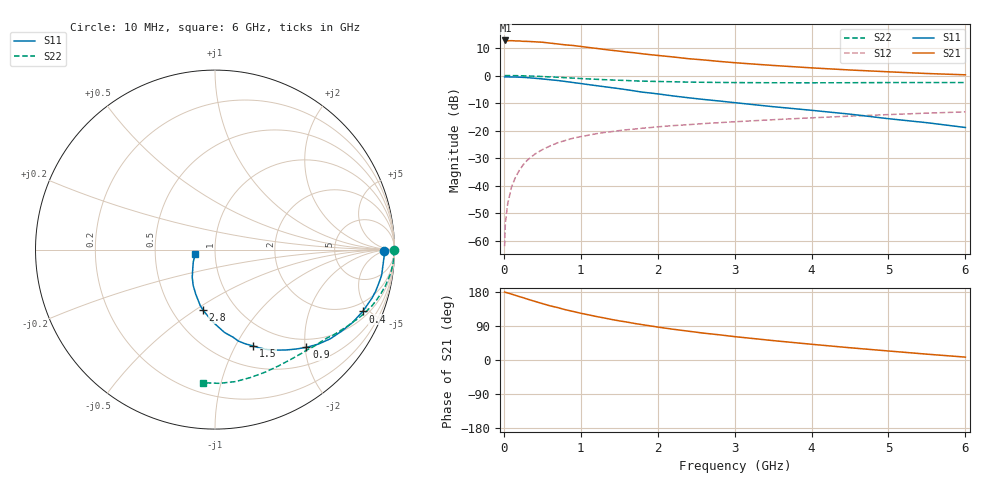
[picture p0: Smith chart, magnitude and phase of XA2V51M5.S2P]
! SIEMENS Discrete & RF Semiconductors
! BFY180
! Si NPN RF Bipolar Junction Transistor in MICRO-X
! VCE = 2.5 V  IC = 1.5 mA
! Common Emitter S-Parameters:  May  1997
# GHz  S  MA  R  50
!  f  S11  S21  S12  S22
! GHz  MAG  ANG  MAG  ANG  MAG  ANG  MAG  ANG
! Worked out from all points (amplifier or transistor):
!   36 points, 10 MHz to 6 GHz, reference 50 ohm
!   highest |S21| = 12.7 dB at 20 MHz (marker M1)
!   |S21| within 3 dB of that: start of sweep to 1.236 GHz
!   unconditionally stable (mu >= 1): 3.09 GHz to end of sweep
!   at 250 MHz: K = 0.11, MSG = 22.4 dB, |S12| = -32.5 dB
!   at 1.4 GHz: K = 0.62, MSG = 14.8 dB, |S12| = -20.4 dB
!   at 6 GHz: K = 1.07, MAG = 5.1 dB, |S12| = -13.2 dB
!   S11 on the Smith chart (normalised r, x): 10 MHz: 33, -5; 400 MHz: 1.36, -4.60; 900 MHz: 0.83, -2.03; 1.5 GHz: 0.73, -1.18; 2.8 GHz: 0.70, -0.54; 6 GHz: 0.80, -0.04
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0.01  0.9422 -0.5  4.269 179.3  0.0008 84.7  0.9964 -0.2
0.02  0.9449 -1.1  4.325 178.6  0.0021 104.7  0.9975 -0.6
0.05  0.9424 -2.7  4.265 177.0  0.0047 88.4  0.996 -1.5
0.1  0.9396 -5.8  4.283 173.9  0.0095 88.2  0.996 -3.1
0.15  0.9395 -8.7  4.247 170.7  0.0141 84.7  0.9945 -4.6
0.25  0.925 -14.4  4.173 164.5  0.0238 80.7  0.9879 -7.6
0.4  0.8925 -22.7  4.093 154.9  0.0372 75.1  0.9711 -11.9
0.5  0.8665 -28.1  4.016 148.9  0.0451 71.5  0.957 -14.7
0.6  0.8387 -32.9  3.872 143.0  0.0526 68.9  0.9438 -17.2
0.8  0.779 -42.6  3.595 132.7  0.0663 62.8  0.9123 -21.9
0.9  0.7458 -46.9  3.506 128.1  0.0728 59.8  0.8971 -24.1
1.1  0.6839 -54.9  3.227 119.2  0.0825 55.6  0.8665 -27.9
1.2  0.6551 -58.7  3.11 114.9  0.0878 53.8  0.8538 -29.8
1.5  0.5775 -68.4  2.768 103.3  0.1001 48.8  0.82 -34.7
1.8  0.4986 -78.3  2.48 93.2  0.1105 45.3  0.7913 -39.1
2.2  0.4258 -88.3  2.171 81.2  0.1232 40.9  0.77 -44.7
2.6  0.3675 -96.9  1.916 70.8  0.1342 37.7  0.7534 -49.9
2.8  0.3447 -101.1  1.802 66.5  0.1395 36.3  0.7479 -52.4
3.5  0.2718 -113.1  1.523 51.2  0.1577 31.2  0.7384 -61.2
4.5  0.199 -129.6  1.259 32.3  0.1832 24.0  0.7395 -74.2
5.5  0.1392 -150.4  1.087 15.4  0.2075 16.4  0.7455 -88.1
6  0.1139 -166.7  1.029 7.6  0.2189 12.3  0.7448 -95.1
